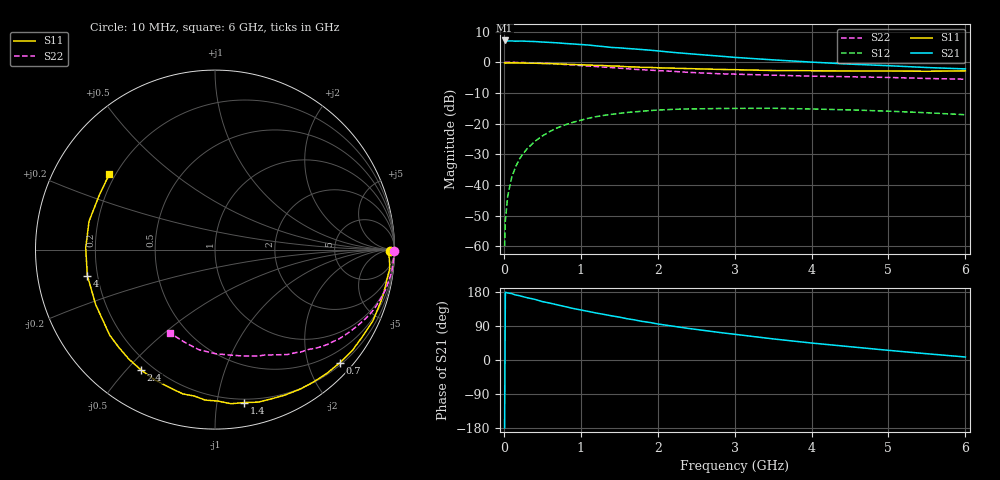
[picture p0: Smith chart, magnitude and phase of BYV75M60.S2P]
! SIEMENS Small Signal Semiconductors
! BFY420
! Si NPN RF SIEGET Grounded Emitter Transistor in MICRO-X
! VCE = 0.75 V  IC = 0.6 mA
! Common Emitter S-Parameters:  October  1996
# GHz  S  MA  R  50
!  f  S11  S21  S12  S22
! GHz  MAG  ANG  MAG  ANG  MAG  ANG  MAG  ANG
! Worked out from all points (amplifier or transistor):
!   36 points, 10 MHz to 6 GHz, reference 50 ohm
!   highest |S21| = 7.1 dB at 10 MHz (marker M1)
!   |S21| within 3 dB of that: start of sweep to 1.811 GHz
!   unconditionally stable (mu >= 1): 4.733 GHz to end of sweep
!   at 250 MHz: K = 0.03, MSG = 18.4 dB, |S12| = -29.8 dB
!   at 1.4 GHz: K = 0.23, MSG = 10.9 dB, |S12| = -17.0 dB
!   at 6 GHz: K = 1.36, MAG = 3.9 dB, |S12| = -17.1 dB
!   S11 on the Smith chart (normalised r, x): 10 MHz: 68, -28; 700 MHz: 0.24, -2.58; 1.4 GHz: 0.17, -1.19; 2.4 GHz: 0.16, -0.55; 4 GHz: 0.16, -0.10; 6 GHz: 0.18, +0.31
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0.01  0.9751 -0.6  2.266 -179.2  0.001 92.4  0.9999 -0.3
0.02  0.9677 -1.3  2.251 178.8  0.0026 99.0  0.9925 -0.7
0.05  0.9734 -3.3  2.222 176.9  0.0065 90.0  0.9987 -1.7
0.1  0.9795 -6.2  2.229 175.4  0.0129 86.1  0.9957 -3.4
0.15  0.9731 -9.2  2.204 171.7  0.0193 83.3  0.9941 -5.0
0.25  0.9702 -15.3  2.213 167.1  0.0322 80.0  0.9887 -8.3
0.4  0.9652 -24.4  2.177 160.2  0.051 73.9  0.9757 -13.3
0.5  0.954 -30.4  2.136 154.2  0.0627 70.2  0.9634 -16.4
0.7  0.9389 -42.1  2.07 145.3  0.0856 62.6  0.936 -22.5
0.9  0.9192 -53.4  1.986 136.0  0.1049 55.0  0.9008 -28.0
1.1  0.8994 -64.3  1.909 128.2  0.1221 48.1  0.867 -33.3
1.4  0.8675 -79.3  1.742 116.6  0.1412 38.7  0.8184 -40.3
1.6  0.8439 -89.0  1.677 109.0  0.1514 32.9  0.7844 -44.5
1.8  0.824 -98.1  1.608 101.8  0.159 27.8  0.7546 -48.1
2.2  0.8002 -114.4  1.447 89.2  0.1704 18.3  0.7103 -55.4
2.4  0.7874 -121.5  1.38 83.3  0.1731 14.6  0.6841 -58.9
2.8  0.764 -134.7  1.26 72.7  0.1761 7.2  0.6491 -64.9
3.5  0.732 -155.3  1.093 55.7  0.1774 -3.1  0.615 -74.7
4  0.7259 -168.5  1.005 44.8  0.1728 -9.4  0.5929 -82.2
4.5  0.7204 179.2  0.931 35.1  0.167 -14.9  0.5796 -90.0
5.5  0.7123 155.2  0.82 16.5  0.1499 -22.8  0.5434 -108.0
6  0.7239 144.4  0.778 7.9  0.1393 -24.7  0.5286 -118.2
